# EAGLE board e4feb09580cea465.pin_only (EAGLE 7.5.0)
DESIGNER: Brent Wilkins; VERSION: v10

Size 17.02 x 17.78 mm. Coordinates in mm from the lower left corner, seen from the top.
Outline: 0,0 10.92,0 10.92,17.78 0,17.78 0,0
Outline: 11.43,0 11.43,17.78 17.02,17.78 17.02,0 11.43,0
Copper layers (1*16): Top 0.035mm / dielectric 1.5mm / Bottom 0.035mm
Design rules "SparkFun-2-layer-FAB-LIMIT": minimum track width 4mil, minimum drill 6mil, track to track 4mil, track to pad 4mil, pad to pad 4mil, via to via 4mil, smd to smd 4mil, copper to edge 4mil, drill to drill 4mil, minimum pad ring 5mil, minimum via ring 5mil, stop-mask expansion 4mil, vias tented up to drill 20mil, thermal gap 10mil

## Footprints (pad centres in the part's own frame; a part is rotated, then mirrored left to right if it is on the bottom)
0603-CAP = smd 1.1 x 1: 1 -0.85,0; 2 0.85,0
FIDUCIAL-1X2 = smd 1 x 1: 1 0,0
1X04 = drill 1.016 pad 1.88 square: 1 0,0 | drill 1.016 pad 1.88: 2 2.54,0; 3 5.08,0; 4 7.62,0
1X03 = drill 1.016 pad 1.88: 1 0,0; 2 2.54,0; 3 5.08,0
0603-RES = smd 1.1 x 1: 1 -0.85,0; 2 0.85,0
PAD-JUMPER-2-NC_BY_PASTE_YES_SILK_FULL_BOX = smd 0.635 x 1.27: 1 -0.412,0; 2 0.412,0
PAD-HUMPER-3-1&2_NC_BY_PASTE_YES_SILK_FULL_BOX = smd 0.635 x 1.27: 1 -0.813,0; 2 0,0; 3 0.813,0
STAND-OFF = hole 3.302: 0,0
QFN24_PAD = smd 0.5 x 0.25: 1 -1.55,1; 2 -1.55,0.6; 3 -1.55,0.2; 4 -1.55,-0.2; 5 -1.55,-0.6; 6 -1.55,-1; 13 1.55,-1; 14 1.55,-0.6; 15 1.55,-0.2; 16 1.55,0.2; 17 1.55,0.6; 18 1.55,1 | smd 0.08 x 0.13: 1$1 -1.32,1.06; 1$3 -1.26,0.94; P$33 1.26,-0.94; P$34 1.32,-1.06; P$58 1.26,0.94; P$59 1.32,1.06; P$68 -1.26,-0.94; P$69 -1.32,-1.06 | smd 0.1 x 0.185 rotated 45: 1$2 -1.25,1.024; P$49 1.024,-1.25 | smd 0.14 x 0.14: 1$4 -1.22,0.945; P$23 -0.945,-1.22; P$24 1.22,-0.945; P$36 0.945,1.22; P$51 0.945,-1.22; P$56 1.22,0.945; P$61 -0.945,1.22; P$66 -1.22,-0.945 | smd 0.05 x 0.05: 1$5 -1.175,0.97; P$25 -0.97,-1.175; P$31 1.175,-0.97; P$37 0.97,1.175; P$52 0.97,-1.175; P$57 1.175,0.97; P$62 -0.97,1.175; P$67 -1.175,-0.97 | smd 0.25 x 0.5: 7 -1,-1.55; 8 -0.6,-1.55; 9 -0.2,-1.55; 10 0.2,-1.55; 11 0.6,-1.55; 12 1,-1.55; 19 1,1.55; 20 0.6,1.55; 21 0.2,1.55; 22 -0.2,1.55; 23 -0.6,1.55; 24 -1,1.55 | smd 0.25 x 0.25: CENTER 0,0 | smd 0.4 x 0.4: DBBADFE -0.675,0.24 | smd 0.6 x 1.2: DBBADFE1 -0.575,-0.195 | smd 0.25 x 0.3: P$1 -0.2,1.3; P$3 0.2,1.3; P$5 0.6,1.3; P$11 -0.6,1.3; P$16 0.2,-1.3; P$18 -0.2,-1.3; P$20 -0.6,-1.3; P$26 0.6,-1.3 | smd 0.3 x 0.25: P$2 -1.3,0.2; P$4 -1.3,0.6; P$28 -1.3,-0.2; P$38 -1.3,-0.6; P$40 1.3,0.2; P$42 1.3,-0.2; P$44 1.3,-0.6; P$50 1.3,0.6 | smd 0.1 x 0.185 rotated 225: P$7 1.25,-1.024; P$60 -1.024,1.25 | smd 1.1 x 1.59: P$13 0.325,0 | smd 0.3 x 0.5 rotated 315: P$14 -0.592,0.512 | smd 0.5 x 1.59: P$15 -0.27,0 | smd 0.1 x 0.185 rotated 135: P$22 -1.024,-1.25; P$55 1.25,1.024 | smd 0.13 x 0.08: P$27 -0.94,-1.26; P$29 -1.06,-1.32; P$39 0.94,1.26; P$41 1.06,1.32; P$53 0.94,-1.26; P$54 1.06,-1.32; P$63 -0.94,1.26; P$64 -1.06,1.32 | smd 0.1 x 0.185 rotated 315: P$35 1.024,1.25; P$65 -1.25,-1.024

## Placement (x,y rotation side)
C1  0.1uF  [0603-CAP]  4.75,4.83 270 top
C2  0.1uF  [0603-CAP]  7.49,8.74 90 top
FID1  FIDUCIAL1X2  [FIDUCIAL-1X2]  10.06,14.48 0 top
FID2  FIDUCIAL1X2  [FIDUCIAL-1X2]  5.82,2.62 0 top
FRAME1  FRAME-LETTER  [CREATIVE_COMMONS]  not placed on the board
J1  [1X04]  2.01,16.51 0 top
J2  [1X03]  9.63,6.35 90 top
J3  [1X04]  2.01,1.27 0 top
LOGO1  SFE_LOGO_FLAME.1_INCH  [SFE_LOGO_FLAME_.1]  15.24,5.08 0 bottom
LOGO2  OSHW-LOGOS  [OSHW-LOGO-S]  14.22,10.41 0 bottom
R1  10K  [0603-RES]  1.93,11.68 180 top
R2  10K  [0603-RES]  1.93,12.95 180 top
R3  10K  [0603-RES]  1.93,14.22 180 top
SJ1  JUMPER-PAD-2-NC_BY_PASTEFULL-BOX-SILK  [PAD-JUMPER-2-NC_BY_PASTE_YES_SILK_FULL_BOX]  1.47,9.47 90 top
SJ2  JUMPER_PAD-3-1&2_NC_BY_PASTE  [PAD-HUMPER-3-1&2_NC_BY_PASTE_YES_SILK_FULL_BOX]  2.01,5.08 180 top
STANDOFF1  STAND-OFF  [STAND-OFF]  14.22,2.79 0 top
STANDOFF2  STAND-OFF  [STAND-OFF]  14.22,14.99 0 top
U1  MPU-9250  [QFN24_PAD]  4.55,8.89 0 top

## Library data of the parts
C1 C2 = SparkFun-Capacitors; PROD_ID: CAP-00810
FID1 FID2 FRAME1 LOGO1 LOGO2 = SparkFun-Aesthetics
J1 J3 = SparkFun-Connectors; PROD_ID: CONN-09696
J2 = SparkFun-Connectors
R1-R3 = SparkFun-Resistors; PROD_ID: RES-00824
SJ1 SJ2 = SparkFun-Passives
STANDOFF1 STANDOFF2 = SparkFun-Electromechanical
U1 = Testing; PROD_ID: IC-13192

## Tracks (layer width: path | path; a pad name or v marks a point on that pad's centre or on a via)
(copper drawn outside any net)
  shapes: Top area x10

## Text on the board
tPlace: MPU-9250 / BREAKOUT | ACCEL & / GRYO | SJ1 | X | Z | Y | MAG | SJ2 | Y | X | Z
bPlace: SCL | SDA | VDD | GND | A&G | AUXDA | Y | X | FSYNC | Z | AUXCL | VDDIO | AD0 / SDO | !CS | INT
Measures: All units in inch
tDocu: V-score for the end user if they want to / remove more than 1/3 of the board size | Don't cut v-score in production!

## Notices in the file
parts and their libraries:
SparkFun-Aesthetics: Licensing: Creative Commons ShareAlike 4.0 International - https://creativecommons.org/licenses/by-sa/4.0
SparkFun-Aesthetics: Released under the Creative Commons Attribution Share-Alike 4.0 License
SparkFun-Aesthetics: https://creativecommons.org/licenses/by-sa/4.0
